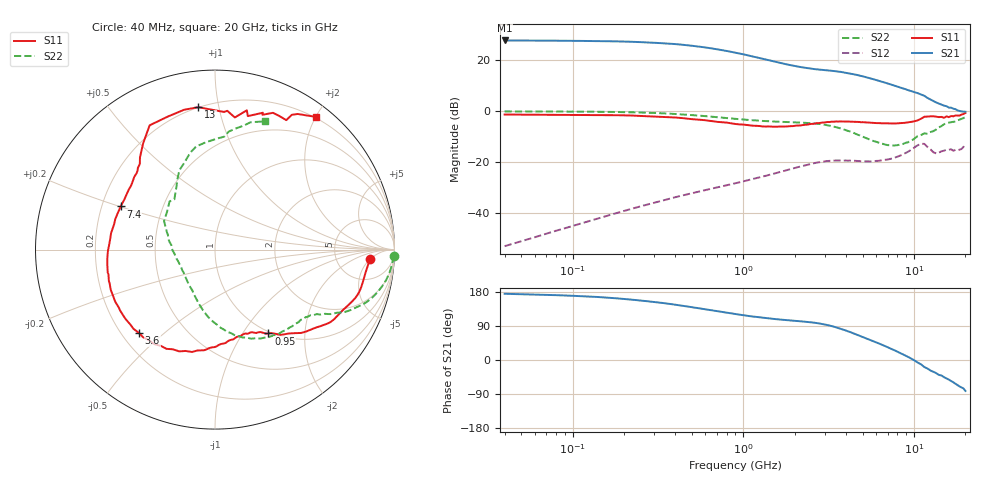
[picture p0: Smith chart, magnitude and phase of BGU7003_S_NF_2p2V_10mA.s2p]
!	Filename:	P:\Prog\Test\Noise\ATS_data\Testdata_Net\BGU7002	BGU7003	RN20082092\BGU7003_B1_high	freq_bias	loop_2.2V9.09mA_D.s2p
!	Date/Time:	Tue	16-Sep-08	9:21:55
!	BGU7003_B1_high	freq_bias	loop
!	bias	mode	1:00	Vout=	2.201	"V,"	Iout=	9.135	"mA,"	Vin=	4.233	"V,"	Iin=	0.978	mA
!	Date/time	Sun	Aug	10	21:21:40	2008
!	Device	data	file	deembeded	for	feedlines	and	parallel
!	Original	file:	\BGU7002	BGU7003	RN20082092\BGU7003_B1_high	freq_bias	loop_2.2V9.09mA_R.s2p
!	Feed-files:	PR029V01_high	"frequency_140808_Feed1.s2p,"	PR029V01_high	frequency_140808_Feed2.s2p
!	Parallel-file:	PR029V01_high	frequency_140808_Par.s2p
#	MHz	S	MA	R	50
!	Freq-MHz	S11-mag	S11-arg	S21-mag	S21-arg	S12-mag	S12-arg	S22-mag	S22-arg
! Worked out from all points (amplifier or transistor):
!   156 points, 40 MHz to 20 GHz, reference 50 ohm
!   highest |S21| = 27.8 dB at 40 MHz (marker M1)
!   |S21| within 3 dB of that: start of sweep to 637 MHz
!   unconditionally stable (mu >= 1): nowhere
!   at 300 MHz: K = 0.24, MSG = 31.4 dB, |S12| = -35.9 dB
!   at 2.15 GHz: K = 0.60, MSG = 19.6 dB, |S12| = -21.7 dB
!   at 20 GHz: K = 0.31, MSG = 7.2 dB, |S12| = -14.5 dB
!   lowest NFmin = 0.55 dB at 400 MHz
!   S11 on the Smith chart (normalised r, x): 40 MHz: 12, -5; 950 MHz: 0.97, -1.31; 3.6 GHz: 0.27, -0.41; 7.4 GHz: 0.28, +0.20; 13 GHz: 0.20, +0.87; 20 GHz: 0.19, +2.00
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40  0.8637 -3.4  24.64 174.8  0.00224 84.4  0.9951 -2.0
80  0.8528 -7.1  24.38 171.1  0.0045 84.5  0.9909 -4.4
120  0.8455 -10.7  24.08 167.9  0.00669 83.7  0.9838 -6.7
190  0.8362 -16.7  23.57 162.0  0.01048 80.8  0.9663 -10.5
230  0.8212 -20.0  23.13 158.6  0.01257 79.1  0.9527 -12.5
320  0.7805 -27.1  21.94 151.7  0.01692 75.9  0.9205 -16.5
410  0.7507 -33.3  20.78 145.2  0.02097 73.0  0.8809 -20.1
550  0.6835 -41.8  18.66 136.4  0.0265 69.7  0.8234 -24.3
700  0.6215 -48.8  16.55 128.8  0.03183 67.1  0.7657 -27.3
900  0.5627 -55.8  14.14 121.1  0.03857 64.9  0.7101 -30.2
950  0.5535 -57.5  13.64 119.7  0.04028 64.5  0.7015 -30.9
1150  0.5194 -62.7  11.83 114.5  0.04691 62.9  0.6662 -32.9
1500  0.4973 -70.1  9.6 108.4  0.05904 59.5  0.6298 -36.7
1950  0.5119 -81.1  7.895 103.8  0.075 54.0  0.6083 -43.0
2600  0.5701 -99.7  6.757 98.5  0.09562 43.2  0.5783 -55.8
3600  0.6288 -132.3  6.021 84.4  0.1079 26.1  0.4737 -79.2
5000  0.6113 -167.9  4.876 61.0  0.104 16.4  0.3186 -105.9
7200  0.5782 157.7  3.424 31.4  0.1154 18.0  0.2157 -147.6
7400  0.5778 155.4  3.321 28.9  0.1177 18.2  0.2128 -152.1
10500  0.662 129.2  2.276 -6.6  0.2145 1.9  0.3253 150.8
13000  0.799 96.6  1.595 -31.1  0.1561 -33.2  0.4081 121.8
20000  0.9281 52.8  0.979 -81.7  0.1884 -61.3  0.7669 68.8
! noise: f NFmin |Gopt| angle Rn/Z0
400  0.554  0.247  9.17  0.124
1000  0.656  0.242  25.4  0.135
1500  0.741  0.24  38.91  0.139
1700  0.776  0.239  44.32  0.14
2200  0.861  0.239  57.84  0.138
3000  0.998  0.243  79.47  0.128
4400  1.237  0.259  117.3  0.1
5800  1.476  0.288  155.2  0.072
8000  1.851  0.36  -159.6  0.065
1.2e+04  2.535  0.571  -112.3  0.357
